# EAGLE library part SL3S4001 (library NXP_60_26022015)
The UHF EPCglobal Generation 2 standard allows the commercialized provision of mass adoption of UHF RFID technology for passive smart tags and labels. Main fields of applications are supply chain management and logistics for worldwide use with special consideration of European, US and Chinese frequencies to ensure that operating distances of several meters can be realized. The UCODE I2C is a product out of the NXP Semiconductors UCODE product family. The entire UCODE product family offers anti-collision and collision arbitration functionality. This allows a reader to simultaneously operate multiple labels/tags within its antenna field. A UCODE I2C based label/ tag requires no external power supply for contactless operation. Its contactless interface generates the power supply via the antenna circuit by propagative energy transmission from the interrogator (reader), while the system clock is generated by an on-chip oscillator. Data transmitted from the interrogator to the label/tag is demodulated by the interface, and it also modulates the interrogator's electromagnetic field for data transmission from the label/tag to the interrogator. A label/tag can be operated without the need for line of sight or battery, as long as it is connected to a dedicated antenna for the targeted frequency range. When the label/tag is within the interrogator's operating range, the high-speed wireless interface allows data transmission in both directions. The UCODE I2C also features an I2C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
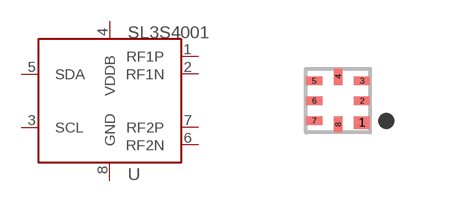
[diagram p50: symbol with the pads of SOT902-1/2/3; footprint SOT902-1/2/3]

Designator prefix U

## SL3S4001  [SOT902-1/2/3]
1  RF1P  pas
2  RF1N  pas
3  SCL
4  VDDB  pwr
5  SDA
6  RF2N  pas
7  RF2P  pas
8  GND  pwr

## Footprint SOT902-1/2/3 (pad centres in mm)
SOT902-1/2/3 XQFN8U: plastic extremely thin quad flat package; no leads; 8 terminals; UTLP based; body 1.6 x 1.6 x 0.5 mm JEDEC: -- IEC: ---
smd 0.4 x 0.32: 1 0.6,-0.55
smd 0.4 x 0.22: 2 0.6,0; 3 0.6,0.5; 5 -0.6,0.5; 6 -0.6,0; 7 -0.6,-0.5
smd 0.22 x 0.4: 4 0,0.6; 8 0,-0.6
